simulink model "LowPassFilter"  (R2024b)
settings: Solver=FixedStepAuto  StartTime=0.0  StopTime=0.3  FixedStep=1e-3  RelTol=1e-3

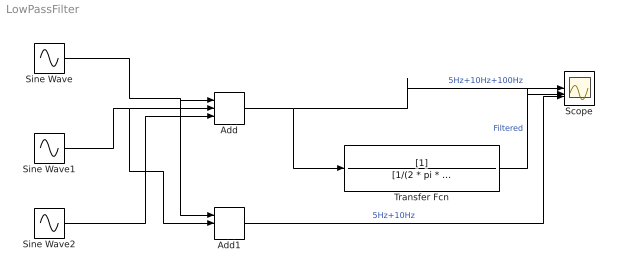
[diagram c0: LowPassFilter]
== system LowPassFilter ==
  Add : Sum  Inputs=+++
  Add1 : Sum  Inputs=+++
  Scope : Scope  NumInputPorts=3
  Sine Wave : Sin  Frequency=2 * pi * 5  SampleTime=0
  Sine Wave1 : Sin  Frequency=2 * pi * 10  Phase=pi/4  SampleTime=0
  Sine Wave2 : Sin  Frequency=2 * pi * 100  Phase=pi/2  SampleTime=0
  Transfer Fcn : TransferFcn  Denominator=[1/(2 * pi * 200) 1]
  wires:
  Sine Wave/1 -> Add1/1, Add/1
  Sine Wave1/1 -> Add1/2, Add/2
  Sine Wave2/1 -> Add/3
  Add/1 -> Transfer Fcn/1, Scope/1  "5Hz+10Hz+100Hz"
  Transfer Fcn/1 -> Scope/2  "Filtered"
  Add1/1 -> Scope/3  "5Hz+10Hz"
